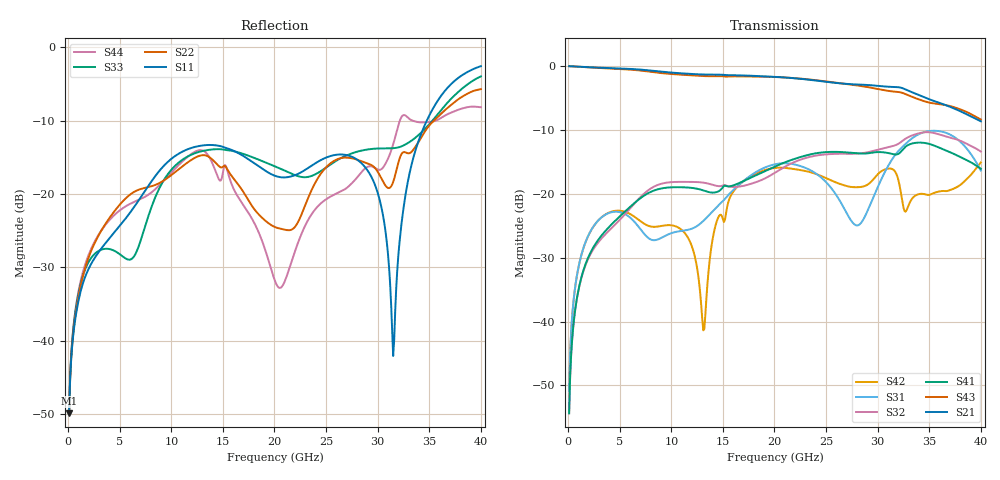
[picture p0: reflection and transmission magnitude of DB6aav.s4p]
! ADC12DJ2700AAV, ADC12DJ3200AAV, ADC08DJ3200AAV
! 144 pin AAV package
! Texas Instruments 4/21/2021
! Single-ended  S-parameters
! PORT#  PORT_NAME  NET_NAME
! PORT1:  DAxN.DIEBUMP DAxN
! PORT2:  DAxN.BGA  DAxN
! PORT3:  DAxP.DIEBUMP DAxP
! PORT4:  DAxP.BGA  DAxP
! Touchstone Ver. 1.0
! Number of ports is 4
# Hz	S	MA	R	50.000000
! SCATTERING PARAMETERS  :
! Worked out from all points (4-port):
!   400 points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, 100 MHz to 40 GHz, reference 50 ohm
!   strongest paths, dB at 100 MHz, 10.1 GHz, 20.1 GHz, 30.1 GHz, 40 GHz:
!     S21: 0.0, -1.0, -1.7, -3.1, -8.6
!     S43: 0.0, -1.3, -1.7, -3.6, -8.4
!     S41: -54.4, -19.0, -15.7, -13.5, -16.1
!     S32: -54.4, -18.2, -16.6, -13.1, -13.4
!     S31: -50.9, -26.1, -15.4, -18.6, -16.4
!     S42: -50.9, -25.0, -15.9, -16.8, -15.1
!   lowest |S11| = -49.9 dB at 100 MHz (marker M1), VSWR 1.01, Z = 50.2 + j0.267 ohm
!   |S11| at or under -10 dB: start of sweep to 34.76 GHz
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1e8  0.003205 56.3  0.9979 -1.4  0.002862 84.8  0.001912 -96.9
     0.9979 -1.4  0.003223 55.1  0.001912 -96.9  0.00286 84.6
     0.002862 84.8  0.001912 -96.9  0.003266 60.2  0.9981 -1.3
     0.001912 -96.9  0.00286 84.6  0.9981 -1.3  0.003271 59.4
3.4e9  0.04419 55.0  0.9682 -43.9  0.06684 38.0  0.04888 -152.3
       0.9682 -43.9  0.05914 -3.0  0.04623 -149.5  0.06703 33.0
       0.06684 38.0  0.04623 -149.5  0.04212 36.9  0.963 -41.3
       0.04888 -152.3  0.06703 33.0  0.963 -41.3  0.05881 4.9
1.28e10  0.2129 -4.2  0.8607 -159.9  0.05831 55.4  0.1082 68.9
         0.8607 -159.9  0.1827 -109.0  0.1231 78.7  0.01674 -72.5
         0.05831 55.4  0.1231 78.7  0.1946 18.3  0.8377 -147.8
         0.1082 68.9  0.01674 -72.5  0.8377 -147.8  0.199 -108.7
2.15e10  0.1311 -41.1  0.8081 91.5  0.1723 21.5  0.1824 -25.8
         0.8081 91.5  0.05674 -98.4  0.171 -4.1  0.1579 -26.2
         0.1723 21.5  0.171 -4.1  0.139 -42.7  0.8094 112.3
         0.1824 -25.8  0.1579 -26.2  0.8094 112.3  0.0321 -69.3
2.93e10  0.1344 -87.9  0.7087 -7.9  0.08309 60.4  0.2089 -142.9
         0.7087 -7.9  0.1586 -104.5  0.2139 -109.3  0.1228 149.5
         0.08309 60.4  0.2139 -109.3  0.2023 -95.8  0.6784 17.4
         0.2089 -142.9  0.1228 149.5  0.6784 17.4  0.1546 -63.3
3.15e10  0.007881 162.3  0.6863 -38.3  0.1914 57.4  0.2044 -174.1
         0.6863 -38.3  0.1208 -72.8  0.2369 -136.9  0.1548 85.0
         0.1914 57.4  0.2369 -136.9  0.2051 -144.2  0.6323 -9.0
         0.2044 -174.1  0.1548 85.0  0.6323 -9.0  0.2178 -43.8
4e10  0.7428 -46.0  0.3694 -150.7  0.1519 -54.3  0.1569 34.9
      0.3694 -150.7  0.518 -101.9  0.214 64.8  0.176 77.3
      0.1519 -54.3  0.214 64.8  0.6326 35.1  0.3817 -110.7
      0.1569 34.9  0.176 77.3  0.3817 -110.7  0.3899 -105.5
